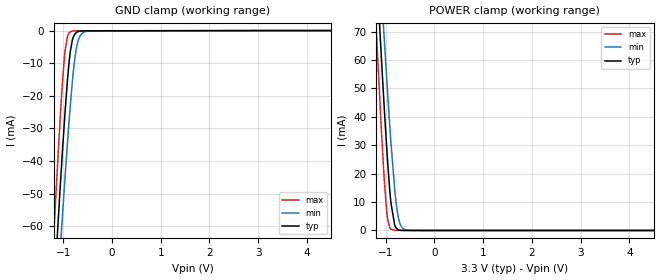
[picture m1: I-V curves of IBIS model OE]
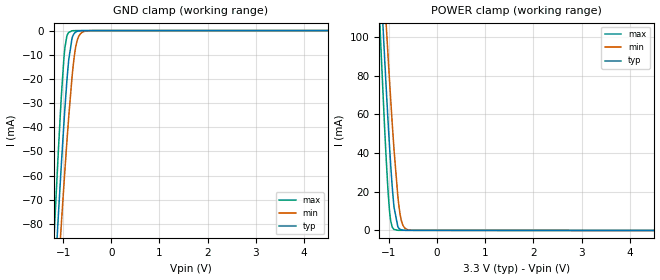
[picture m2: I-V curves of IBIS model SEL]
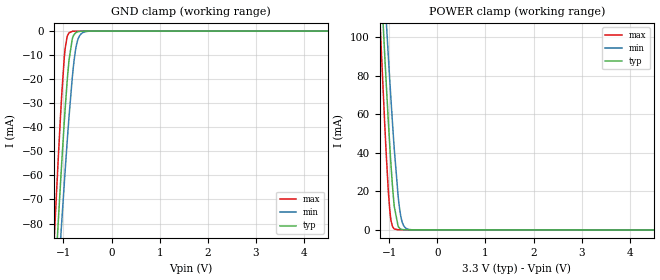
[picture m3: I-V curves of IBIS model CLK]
| Texas Instruments Incorporated
| Low Skew, 1-to-5, Differential-to-3.3V LVPECL Fanout Buffer
| Marketing part#   Voltage Range   Package-type   #pins/pkg drawing
| LMK00804BPW   1.425V - 3.465V   TSSOP   20/PW
[IBIS Ver]   4.1
[File name]   lmk00804.ibs
[File Rev]   1.1
[Date]   01/20/2015
[Source]   Model built from spectre simulations at:
   Texas Instruments Incorporated.
   Analog-eLab, HPA
   12500 TI Blvd
   Dallas, TX -75243
   For Support e-mail: elab_ibis@list.ti.com
[Notes]   Revision History
   Rev 1.1: 01/20/2015
   - Update LVCMOS_CLK, OE, CLK models
   Rev 1.0: 06/27/2014
   - ccomp values are based on PVT settings:
   MIN: Low Voltage, High Temperature, Weak Process
   TYP: Nominal Voltage, Nominal Temperature, Nominal Process
   MAX: High Voltage, Low Temperature, Fast Process
   - C_comp although listed in numerical order of value are obtained from varying PVT conditions.
   For PVT conditions for each specific value, refer to the buffer description under respective [Model].
   IBIS model user is responsible for using appropriate C_comp to simulate for Signal Integrity.
[Disclaimer]  This model is designed as an aid for customers of Texas Instruments
 TI and its licensors and suppliers make no warranties, either expressed
 or implied, with respect to this  model, including the warranties of
 merchantability or fitness for a particular purpose.
 The model is provided solely on an "as is" basis. The entire risk as to
 its quality and performance is with the customer.
[Copyright] (C)Copyright 2014 Texas Instruments Incorporated.
   All rights reserved.
[Component]   LMK00804BPW
[Manufacturer]  Texas Instruments Incorporated
[Package]   |16-pin TSSOP PW package
|   typ   min   max
R_pkg   0.3009   0.1896   0.3774
L_pkg   2.4949n   1.8987n   3.1614n
C_pkg   0.355p   0.2832p   0.4988p
[Pin]   signal_name   model_name   R_pin   L_pin   C_pin
1   GND   GND   0.31653  3.14288n  0.45390p
2   OE   OE   0.37741  3.16140n  0.42943p
3   VCC   POWER   0.34370  2.47224n  0.32523p
4   CLK_EN   OE   0.28830  2.13486n  0.30232p
5   CLK   CLK   0.24981  1.90327n  0.28534p
6   nCLK   CLK   0.24988  1.90366n  0.28537p
7   CLK_SEL   SEL   0.28844  2.13574n  0.30240p
8   LVCMOS_CLK   LVCMOS_CLK   0.34390  2.47345n  0.32530p
9   GND   GND   0.37729  3.15779n  0.43025p
10   Q3   QOUT   0.31651  3.14242n  0.45386p
11   VDD0   POWER   0.18956  2.90445n  0.49875p
12   Q2   QOUT   0.35667  3.03990n  0.41819p
13   GND   GND   0.32975  2.39344n  0.31031p
14   Q1   QOUT   0.28522  2.12364n  0.29683p
15   VDD0   POWER   0.25309  1.93124n  0.28500p
16   Q0   QOUT   0.24763  1.89871n  0.28319p
[Diff pin]  inv_pin  vdiff  tdelay_typ  tdelay_min  tdelay_max
5   6   0.15   NA   NA   NA
[Model Selector] QOUT
QOUT_3P3V   Qn output, 3.3V supply
QOUT_2P5V   Qn output, 2.5V supply
QOUT_1P8V   Qn output, 1.8V supply
QOUT_1P5V   Qn output, 1.5V supply
| Models and submodels in the file (8): OE (Input), SEL (Input), CLK (Input), LVCMOS_CLK (Input), QOUT_3P3V (3-state), QOUT_2P5V (3-state), QOUT_1P8V (3-state), QOUT_1P5V (3-state)
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|   Model OE
[Model]   OE
Model_type   Input
Vinl = .8
Vinh = 2
|   typ   min   max
|   (nom PVT)   (fast PVT)   (slow PVT)
C_comp   0.309p   0.301p   0.316p
[Voltage Range]   3.3   3.135   3.465
[Temperature Range]   45   125   -40
[Power Clamp Reference]   3.3   3.135   3.465
[GND Clamp Reference]   0   0   0
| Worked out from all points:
|   GND clamp passes 1 mA (typ) near -0.76 V on its own axis
|   POWER clamp passes 1 mA (typ) near -0.79 V on its own axis
[GND Clamp]
|   Voltage   I(typ)   I(min)   I(max)
-3.3V     -663.9mA   -633.4mA   -705.9mA
-1.191V   -80.45mA   -97.56mA   -61.59mA
-1.102V   -57.74mA   -76.43mA   -36.99mA
-1.033V   -40.8mA    -60.42mA   -19.52mA
-963.6mV  -25.06mA   -44.98mA   -6.122mA
-914.1mV  -15.2mA    -34.49mA   -1.758mA
-854.7mV  -6.334mA   -22.85mA   -386.1uA
-785.4mV  -1.697mA   -11.53mA   -105.2uA
-716.1mV  -459.5uA   -4.373mA   -83.65uA
-636.9mV  -127.4uA   -1.282mA   -81.35uA
-518.1mV  -76.95uA   -218.7uA   -78.98uA
6.6V      0A         0A         0A
[POWER Clamp]
|   Voltage   I(typ)   I(min)   I(max)
-3.3V     825.2mA    793.2mA    869.6mA
-1.201V   96.02mA    117.6mA    72.91mA
-1.171V   86.44mA    108.6mA    62.56mA
-1.092V   61.5mA     85.09mA    36.13mA
-1.033V   43.68mA    67.95mA    18.46mA
-963.6mV  24.68mA    48.78mA    4.242mA
-894.3mV  9.716mA    31.06mA    452.1uA
-815.1mV  1.765mA    14.2mA     29.45uA
-755.7mV  397.1uA    5.855mA    15.68uA
-686.4mV  55.73uA    1.605mA    13.63uA
-587.4mV  12.9uA     196uA      11.64uA
6.6V      0A         0A         0A
|   Model SEL
[Model]   SEL
Model_type   Input
Vinl = .8
Vinh = 2
|   typ   min   max
|   (nom PVT)   (fast PVT)   (slow PVT)
C_comp   0.309p   0.301p   0.316p
[Voltage Range]   3.3   3.135   3.465
[Temperature Range]   45   125   -40
[Power Clamp Reference]   3.3   3.135   3.465
[GND Clamp Reference]   0   0   0
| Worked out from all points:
|   GND clamp passes 1 mA (typ) near -0.76 V on its own axis
|   POWER clamp passes 1 mA (typ) near -0.79 V on its own axis
[GND Clamp]
|   Voltage   I(typ)   I(min)   I(max)
-3.3V     -924.2mA   -854.8mA   -1.024A
-1.181V   -105.5mA   -125.5mA   -82.35mA
-1.102V   -77.37mA   -100.2mA   -50.77mA
-1.043V   -57.12mA   -81.6mA    -29mA
-973.5mV  -35.04mA   -60.66mA   -9.026mA
-924mV    -21.16mA   -46.42mA   -2.356mA
-884.4mV  -12.1mA    -35.68mA   -770.7uA
-815.1mV  -3.137mA   -19.14mA   -90.22uA
-755.7mV  -921.7uA   -8.805mA   -20.2uA
-706.2mV  -319uA     -3.926mA   -14.46uA
-508.2mV  -10.71uA   -130.8uA   -10.08uA
6.6V      0A         0A         0A
[POWER Clamp]
|   Voltage   I(typ)   I(min)   I(max)
-3.3V     1.278A     1.181A     1.417A
-1.191V   138.4mA    165.4mA    108mA
-1.181V   133.4mA    160.9mA    102.4mA
-1.092V   89.93mA    121.4mA    53.98mA
-1.063V   76mA       108.5mA    39.24mA
-983.4mV  41.38mA    75.41mA    8.902mA
-894.3mV  11.89mA    41.49mA    528.2uA
-815.1mV  1.91mA     17.52mA    98.21uA
-765.6mV  589.4uA    7.921mA    85.08uA
-706.2mV  163uA      2.529mA    82.81uA
-597.3mV  79.45uA    310.2uA    80.59uA
6.6V      0A         0A         0A
|   Model CLK
[Model]   CLK
Model_type   Input
Vinl = 1.2
Vinh = 1.5
|   typ   min   max
|   (nom PVT)   (fast PVT)   (slow PVT)
C_comp   0.309p   0.301p   0.316p
[Voltage Range]   3.3   3.135   3.465
[Temperature Range]   45   125   -40
[Power Clamp Reference]   3.3   3.135   3.465
[GND Clamp Reference]   0   0   0
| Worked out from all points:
|   GND clamp passes 1 mA (typ) near -0.76 V on its own axis
|   POWER clamp passes 1 mA (typ) near -0.79 V on its own axis
[GND Clamp]
|   Voltage   I(typ)   I(min)   I(max)
-3.3V     -924.2mA   -854.8mA   -1.024A
-1.181V   -105.5mA   -125.5mA   -82.35mA
-1.102V   -77.37mA   -100.2mA   -50.77mA
-1.043V   -57.12mA   -81.6mA    -29mA
-973.5mV  -35.04mA   -60.66mA   -9.026mA
-924mV    -21.16mA   -46.42mA   -2.356mA
-884.4mV  -12.1mA    -35.68mA   -770.7uA
-815.1mV  -3.137mA   -19.14mA   -90.22uA
-755.7mV  -921.7uA   -8.805mA   -20.2uA
-706.2mV  -319uA     -3.926mA   -14.46uA
-508.2mV  -10.71uA   -130.8uA   -10.08uA
6.6V      0A         0A         0A
[POWER Clamp]
|   Voltage   I(typ)   I(min)   I(max)
-3.3V     1.278A     1.181A     1.417A
-1.191V   138.4mA    165.4mA    108mA
-1.181V   133.4mA    160.9mA    102.4mA
-1.092V   89.93mA    121.4mA    53.98mA
-1.063V   76mA       108.5mA    39.24mA
-983.4mV  41.38mA    75.41mA    8.902mA
-894.3mV  11.89mA    41.49mA    528.2uA
-815.1mV  1.91mA     17.52mA    98.21uA
-765.6mV  589.4uA    7.921mA    85.08uA
-706.2mV  163uA      2.529mA    82.81uA
-597.3mV  79.45uA    310.2uA    80.59uA
6.6V      0A         0A         0A
